(* Logix 5000 Routine export Unit1_Sample; software revision 20.05 *)

TYPE Unit_Type :   // Common information for a unit
STRUCT
   Alm_Reset : BOOL;   // Alarm reset
   Local : BOOL;   // Local/remote control indication
   Maint : BOOL;   // Maintenance privilege for device control
   Man_StartOpen : BOOL;   // Manual start/open from operator
   Man_StopClose : BOOL;   // Manual stop/close from operator
   Man_DevNum : DINT;   // Number of device started/stopped at OI
   Msg : DINT;   // Message number
   Time_Remaining : DINT;   // Remaining time in timed steps
END_STRUCT
END_TYPE

TYPE Seq_Type :   // Sequence Information
STRUCT
   Step_Num : DINT;   // Current step number
   Running : BOOL;   // Running indication
   PC_Start : BOOL;   // Sequence start request from PC
   LTP_Start : BOOL;   // Sequence start request from LTP
   Ons : BOOL;   // One-shot storage to start
   Auto_Start : BOOL;   // Auto-start request
   Auto_Ons : BOOL;   // Auto-start one-shot storage
   Req_Tmr : TIMER;   // Auto-start hold timer
END_STRUCT
END_TYPE

VAR_GLOBAL   (* controller tags *)
   Unit1_Hold : Seq_Type := (Req_Tmr.PRE := 5000);   // Unit Desc1 Hold Sequence
   Unit1_Sample : Seq_Type := (Req_Tmr.PRE := 5000);   // Unit Desc1 Sample Sequence
   Unit1 : Unit_Type;   // Unit Desc1
   Unit1_Shutdown : Seq_Type := (Req_Tmr.PRE := 5000);   // Unit Desc1 Shutdown Sequence
   Unit1_Eshutdown : Seq_Type := (Req_Tmr.PRE := 5000);   // Unit Desc1 E-Shutdown Sequence
END_VAR

PROGRAM MainProgram

ROUTINE Unit1_Sample   (* ladder *)
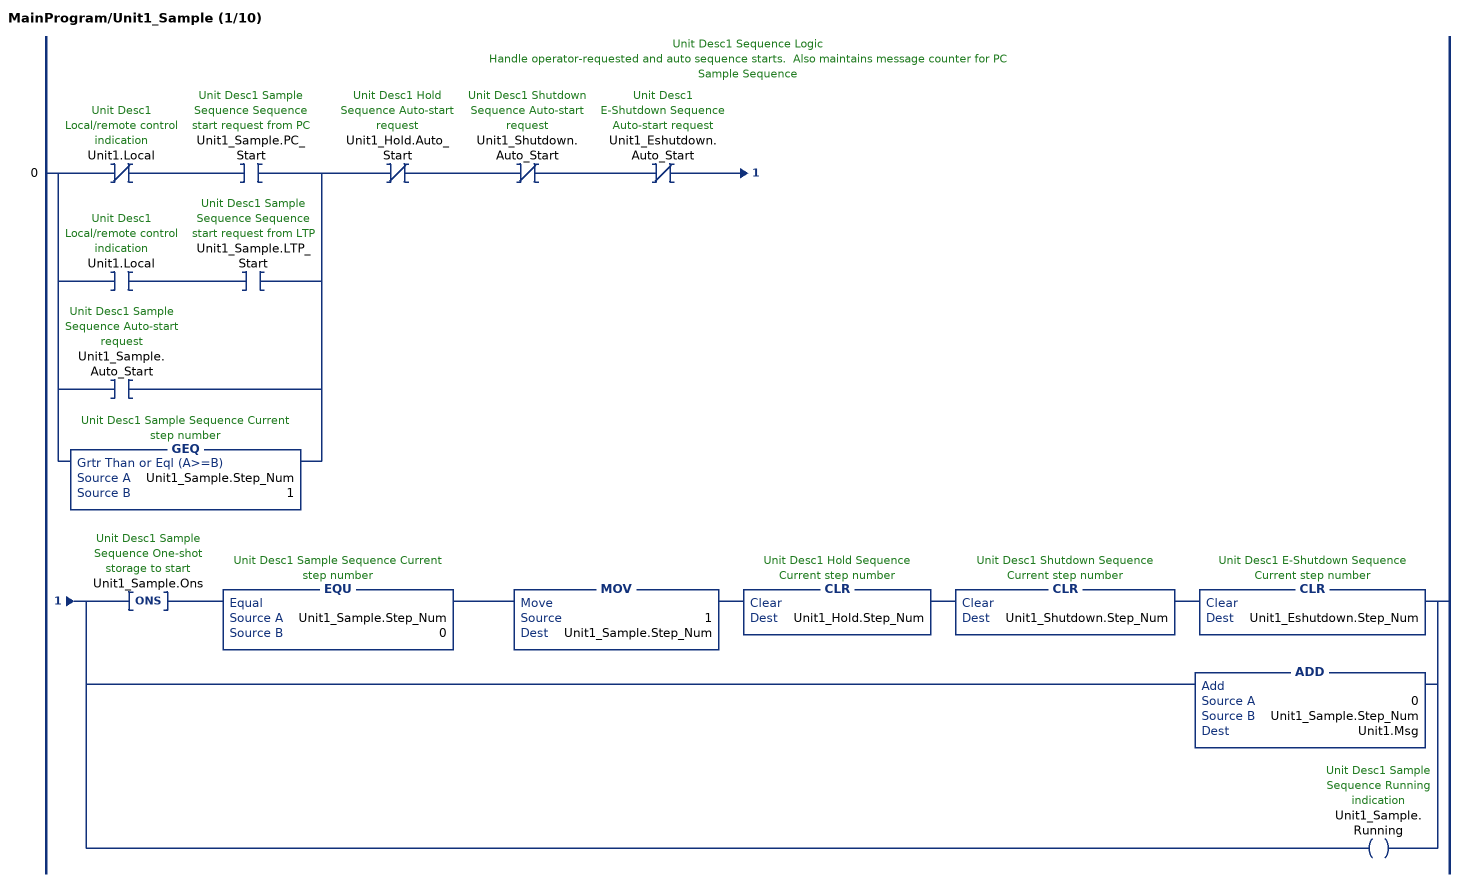
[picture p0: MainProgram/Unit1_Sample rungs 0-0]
   // Unit Desc1 Sequence Logic
   // Handle operator-requested and auto sequence starts.  Also maintains message counter for PC
   // Sample Sequence
   0: [XIO(Unit1.Local) XIC(Unit1_Sample.PC_Start) ,XIC(Unit1.Local) XIC(Unit1_Sample.LTP_Start) ,XIC(Unit1_Sample.Auto_Start) ,GEQ(Unit1_Sample.Step_Num,1) ]XIO(Unit1_Hold.Auto_Start)XIO(Unit1_Shutdown.Auto_Start)XIO(Unit1_Eshutdown.Auto_Start)[ONS(Unit1_Sample.Ons) EQU(Unit1_Sample.Step_Num,0) MOV(1,Unit1_Sample.Step_Num) CLR(Unit1_Hold.Step_Num) CLR(Unit1_Shutdown.Step_Num) CLR(Unit1_Eshutdown.Step_Num) ,ADD(0,Unit1_Sample.Step_Num,Unit1.Msg) ,OTE(Unit1_Sample.Running) ];
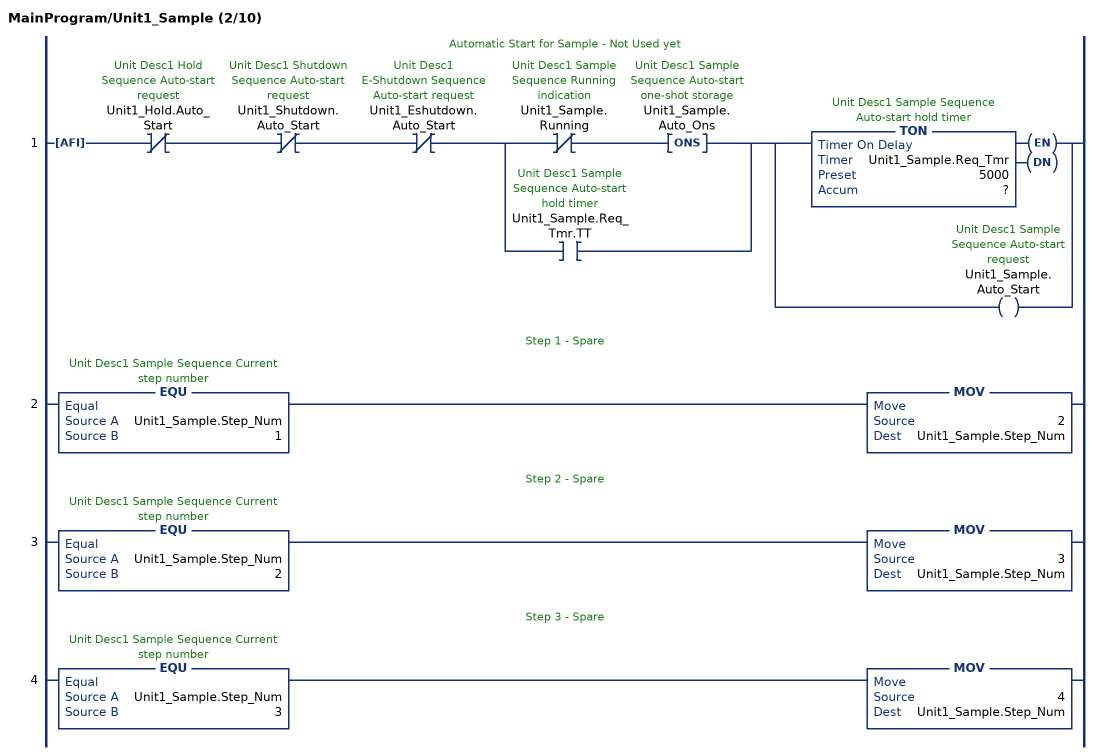
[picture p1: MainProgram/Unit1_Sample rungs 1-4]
   // Automatic Start for Sample - Not Used yet
   1: AFI()XIO(Unit1_Hold.Auto_Start)XIO(Unit1_Shutdown.Auto_Start)XIO(Unit1_Eshutdown.Auto_Start)[XIO(Unit1_Sample.Running) ONS(Unit1_Sample.Auto_Ons) ,XIC(Unit1_Sample.Req_Tmr.TT) ][TON(Unit1_Sample.Req_Tmr,?,?) ,OTE(Unit1_Sample.Auto_Start) ];
   // Step 1 - Spare
   2: EQU(Unit1_Sample.Step_Num,1)MOV(2,Unit1_Sample.Step_Num);
   // Step 2 - Spare
   3: EQU(Unit1_Sample.Step_Num,2)MOV(3,Unit1_Sample.Step_Num);
   // Step 3 - Spare
   4: EQU(Unit1_Sample.Step_Num,3)MOV(4,Unit1_Sample.Step_Num);
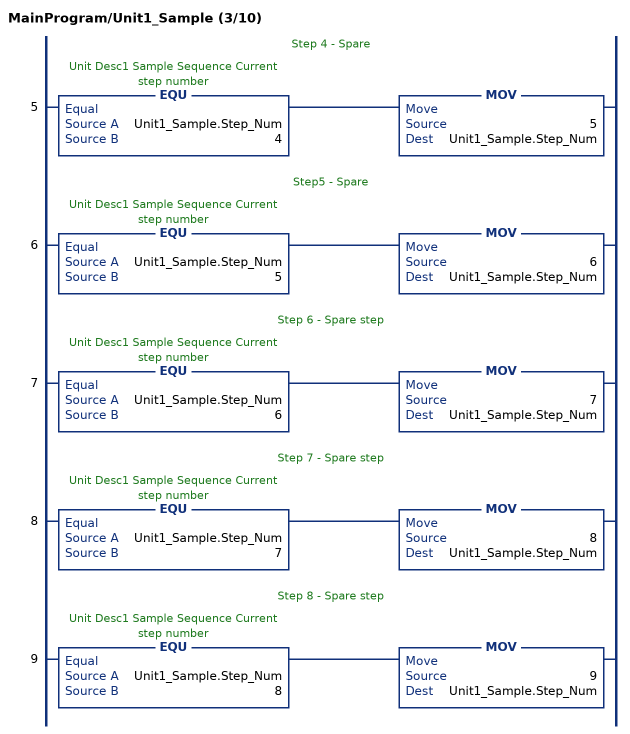
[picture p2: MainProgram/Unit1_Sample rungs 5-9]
   // Step 4 - Spare
   5: EQU(Unit1_Sample.Step_Num,4)MOV(5,Unit1_Sample.Step_Num);
   // Step5 - Spare
   6: EQU(Unit1_Sample.Step_Num,5)MOV(6,Unit1_Sample.Step_Num);
   // Step 6 - Spare step
   7: EQU(Unit1_Sample.Step_Num,6)MOV(7,Unit1_Sample.Step_Num);
   // Step 7 - Spare step
   8: EQU(Unit1_Sample.Step_Num,7)MOV(8,Unit1_Sample.Step_Num);
   // Step 8 - Spare step
   9: EQU(Unit1_Sample.Step_Num,8)MOV(9,Unit1_Sample.Step_Num);
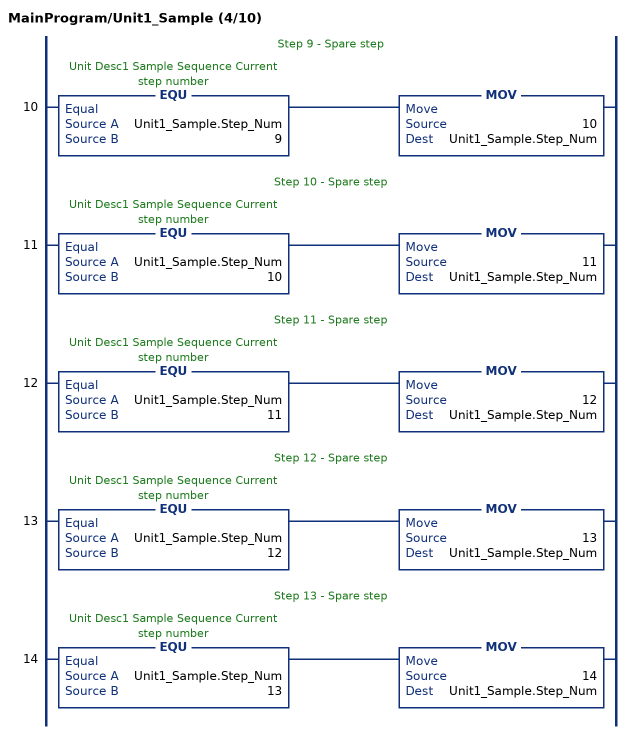
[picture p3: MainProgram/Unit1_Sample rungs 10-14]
   // Step 9 - Spare step
   10: EQU(Unit1_Sample.Step_Num,9)MOV(10,Unit1_Sample.Step_Num);
   // Step 10 - Spare step
   11: EQU(Unit1_Sample.Step_Num,10)MOV(11,Unit1_Sample.Step_Num);
   // Step 11 - Spare step
   12: EQU(Unit1_Sample.Step_Num,11)MOV(12,Unit1_Sample.Step_Num);
   // Step 12 - Spare step
   13: EQU(Unit1_Sample.Step_Num,12)MOV(13,Unit1_Sample.Step_Num);
   // Step 13 - Spare step
   14: EQU(Unit1_Sample.Step_Num,13)MOV(14,Unit1_Sample.Step_Num);
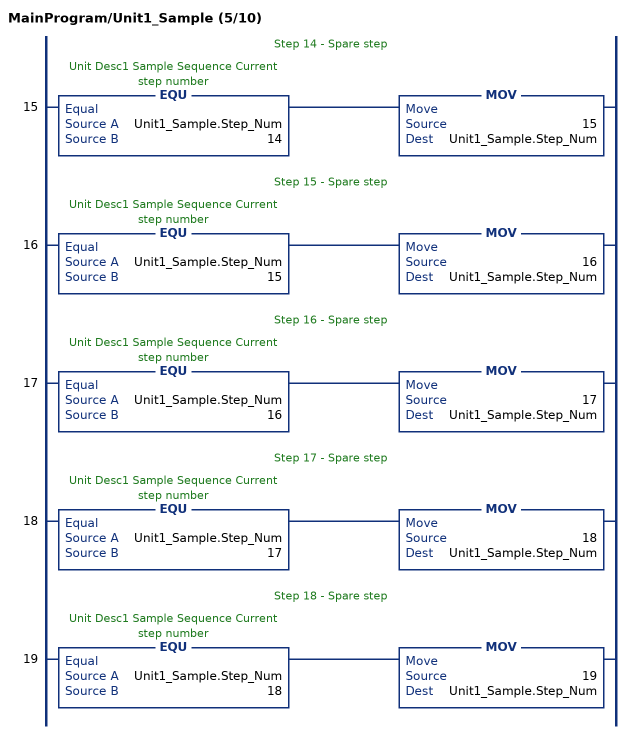
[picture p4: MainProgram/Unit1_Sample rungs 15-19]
   // Step 14 - Spare step
   15: EQU(Unit1_Sample.Step_Num,14)MOV(15,Unit1_Sample.Step_Num);
   // Step 15 - Spare step
   16: EQU(Unit1_Sample.Step_Num,15)MOV(16,Unit1_Sample.Step_Num);
   // Step 16 - Spare step
   17: EQU(Unit1_Sample.Step_Num,16)MOV(17,Unit1_Sample.Step_Num);
   // Step 17 - Spare step
   18: EQU(Unit1_Sample.Step_Num,17)MOV(18,Unit1_Sample.Step_Num);
   // Step 18 - Spare step
   19: EQU(Unit1_Sample.Step_Num,18)MOV(19,Unit1_Sample.Step_Num);
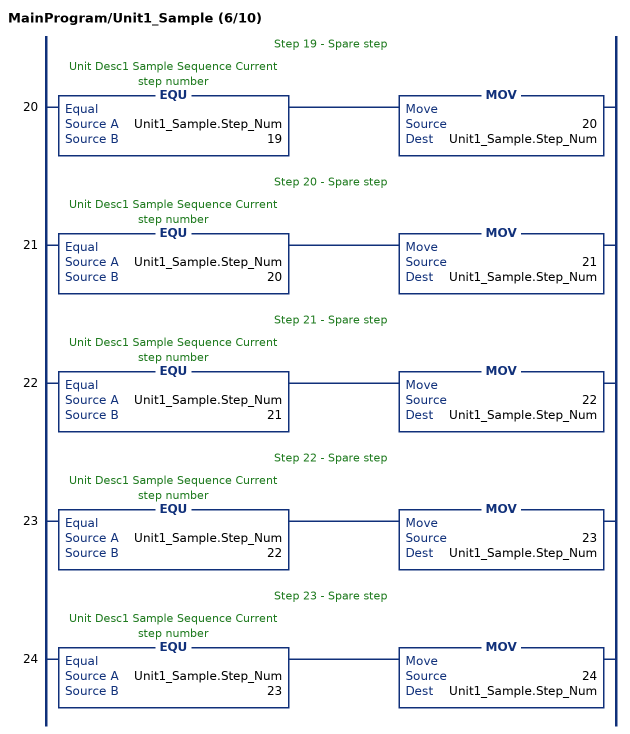
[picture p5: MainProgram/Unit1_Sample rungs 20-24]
   // Step 19 - Spare step
   20: EQU(Unit1_Sample.Step_Num,19)MOV(20,Unit1_Sample.Step_Num);
   // Step 20 - Spare step
   21: EQU(Unit1_Sample.Step_Num,20)MOV(21,Unit1_Sample.Step_Num);
   // Step 21 - Spare step
   22: EQU(Unit1_Sample.Step_Num,21)MOV(22,Unit1_Sample.Step_Num);
   // Step 22 - Spare step
   23: EQU(Unit1_Sample.Step_Num,22)MOV(23,Unit1_Sample.Step_Num);
   // Step 23 - Spare step
   24: EQU(Unit1_Sample.Step_Num,23)MOV(24,Unit1_Sample.Step_Num);
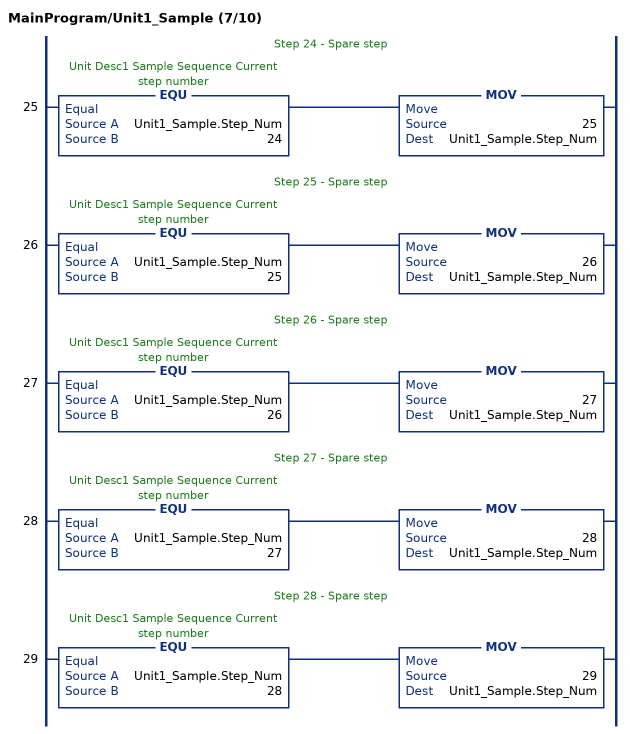
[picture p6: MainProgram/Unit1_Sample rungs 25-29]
   // Step 24 - Spare step
   25: EQU(Unit1_Sample.Step_Num,24)MOV(25,Unit1_Sample.Step_Num);
   // Step 25 - Spare step
   26: EQU(Unit1_Sample.Step_Num,25)MOV(26,Unit1_Sample.Step_Num);
   // Step 26 - Spare step
   27: EQU(Unit1_Sample.Step_Num,26)MOV(27,Unit1_Sample.Step_Num);
   // Step 27 - Spare step
   28: EQU(Unit1_Sample.Step_Num,27)MOV(28,Unit1_Sample.Step_Num);
   // Step 28 - Spare step
   29: EQU(Unit1_Sample.Step_Num,28)MOV(29,Unit1_Sample.Step_Num);
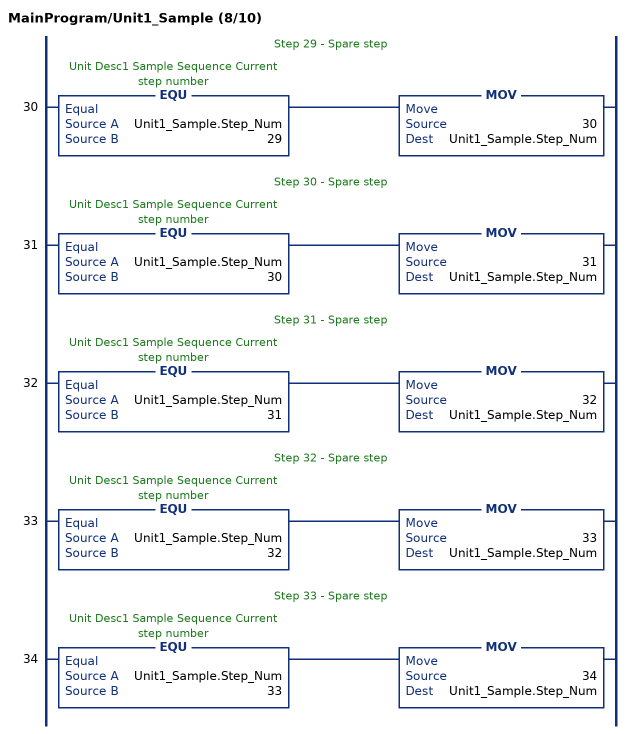
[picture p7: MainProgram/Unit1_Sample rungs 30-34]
   // Step 29 - Spare step
   30: EQU(Unit1_Sample.Step_Num,29)MOV(30,Unit1_Sample.Step_Num);
   // Step 30 - Spare step
   31: EQU(Unit1_Sample.Step_Num,30)MOV(31,Unit1_Sample.Step_Num);
   // Step 31 - Spare step
   32: EQU(Unit1_Sample.Step_Num,31)MOV(32,Unit1_Sample.Step_Num);
   // Step 32 - Spare step
   33: EQU(Unit1_Sample.Step_Num,32)MOV(33,Unit1_Sample.Step_Num);
   // Step 33 - Spare step
   34: EQU(Unit1_Sample.Step_Num,33)MOV(34,Unit1_Sample.Step_Num);
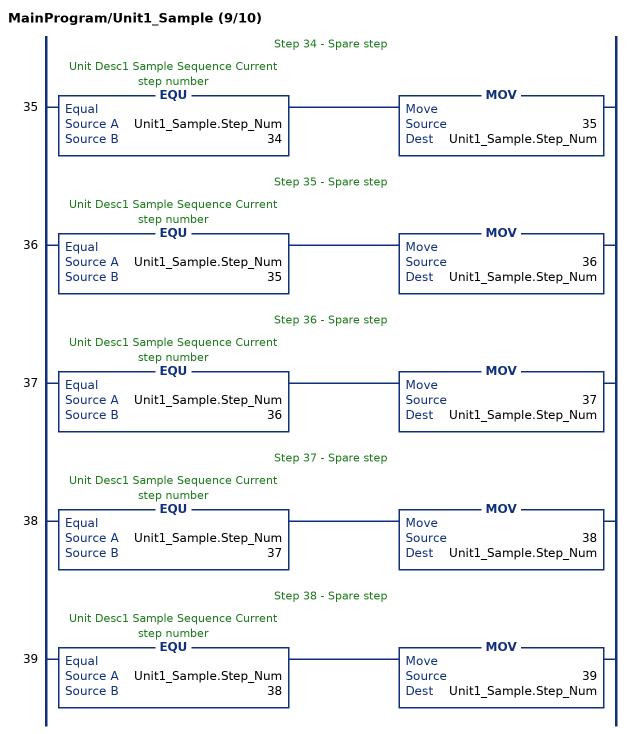
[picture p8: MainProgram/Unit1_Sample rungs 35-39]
   // Step 34 - Spare step
   35: EQU(Unit1_Sample.Step_Num,34)MOV(35,Unit1_Sample.Step_Num);
   // Step 35 - Spare step
   36: EQU(Unit1_Sample.Step_Num,35)MOV(36,Unit1_Sample.Step_Num);
   // Step 36 - Spare step
   37: EQU(Unit1_Sample.Step_Num,36)MOV(37,Unit1_Sample.Step_Num);
   // Step 37 - Spare step
   38: EQU(Unit1_Sample.Step_Num,37)MOV(38,Unit1_Sample.Step_Num);
   // Step 38 - Spare step
   39: EQU(Unit1_Sample.Step_Num,38)MOV(39,Unit1_Sample.Step_Num);
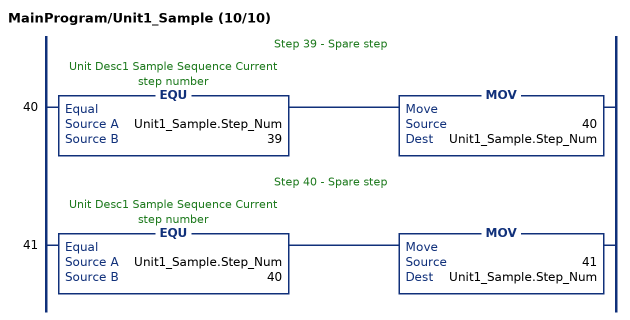
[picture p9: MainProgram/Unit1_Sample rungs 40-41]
   // Step 39 - Spare step
   40: EQU(Unit1_Sample.Step_Num,39)MOV(40,Unit1_Sample.Step_Num);
   // Step 40 - Spare step
   41: EQU(Unit1_Sample.Step_Num,40)MOV(41,Unit1_Sample.Step_Num);
END_ROUTINE
END_PROGRAM
